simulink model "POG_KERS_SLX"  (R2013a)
settings: Solver=ode45  StartTime=0.0  StopTime=10.0  MaxStep=0.001  RelTol=1e-3
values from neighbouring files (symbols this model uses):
  b_1 = 0    [POG_KERS_Par_SLX_m.m]    (also in POG_KERS_SLX_m.m = 1)
  b_2 = 0    [POG_KERS_Par_SLX_m.m]    (also in POG_KERS_SLX_m.m = 1)
  b_3 = 0    [POG_KERS_Par_SLX_m.m]    (also in POG_KERS_SLX_m.m = 1)
  b_b = 0    [POG_KERS_Par_SLX_m.m]    (also in POG_KERS_SLX_m.m = 1)
  J_1 = 0.026*kg*meters^2    [POG_KERS_Par_SLX_m.m]    (also in POG_KERS_SLX_m.m = 13)
  J_2 = 0.675*kg*r_2^2    [POG_KERS_Par_SLX_m.m]    (also in POG_KERS_SLX_m.m = 1)
  J_3 = 100*J_2    [POG_KERS_Par_SLX_m.m]    (also in POG_KERS_SLX_m.m = 1)
  J_b = 1.0*kg*r_b^2    [POG_KERS_Par_SLX_m.m]    (also in POG_KERS_SLX_m.m = 1)
  K_1_2 = Inf    (= inf)    [POG_KERS_EQN_Reduced.m]    (also in POG_KERS_Par_SLX_m.m = 150*Newton/(0.2*mm); POG_KERS_SLX_m.m = 1)
  K_2_b = Inf    (= inf)    [POG_KERS_EQN_Reduced.m]    (also in POG_KERS_Par_SLX_m.m = 80*Newton/(0.2*mm); POG_KERS_SLX_m.m = 1)
  K_b_3 = Inf    (= inf)    [POG_KERS_EQN_Reduced.m]    (also in POG_KERS_Par_SLX_m.m = 80*Newton/(0.2*mm); POG_KERS_SLX_m.m = 1)
  P_1_6_0 = 0    [POG_KERS_SLX_m.m]
  P_2_0 = 2    [POG_KERS_SLX_m.m]
  P_2_3_0 = 0    [POG_KERS_SLX_m.m]
  P_9_0 = 0    [POG_KERS_SLX_m.m]
  r_1 = 17.2*mm    [POG_KERS_Par_SLX_m.m]    (also in POG_KERS_SLX_m.m = 1)
  r_2 = 51.5*mm    [POG_KERS_Par_SLX_m.m]    (also in POG_KERS_SLX_m.m = 1)
  r_2_t_h = r_a+r_b*sin(th_0)    [POG_KERS_Par_SLX_m.m]    (also in POG_KERS_SLX_m.m = 1)
  r_3_t_h = r_a-r_b*sin(th_0)    [POG_KERS_Par_SLX_m.m]    (also in POG_KERS_SLX_m.m = 1)
  r_b = 27.5*mm    [POG_KERS_Par_SLX_m.m]    (also in POG_KERS_SLX_m.m = 1)
  T_1_0 = 0*Nm    [POG_KERS_Par_SLX_m.m]    (also in POG_KERS_SLX_m.m = 0)
  Ts = Tfin/Nr_Ts_Points    (= 0.0015)    [POG_KERS_Par_SLX_m.m]    (also in POG_KERS_SLX_m.m = 0.005)
  x_1_3_0 = 0    [POG_KERS_Par_SLX_m.m]    (also in POG_KERS_SLX_m.m)
  x_2_0_0 = 0    [POG_KERS_Par_SLX_m.m]    (also in POG_KERS_SLX_m.m)
  x_6_0 = 0    [POG_KERS_Par_SLX_m.m]    (also in POG_KERS_SLX_m.m)

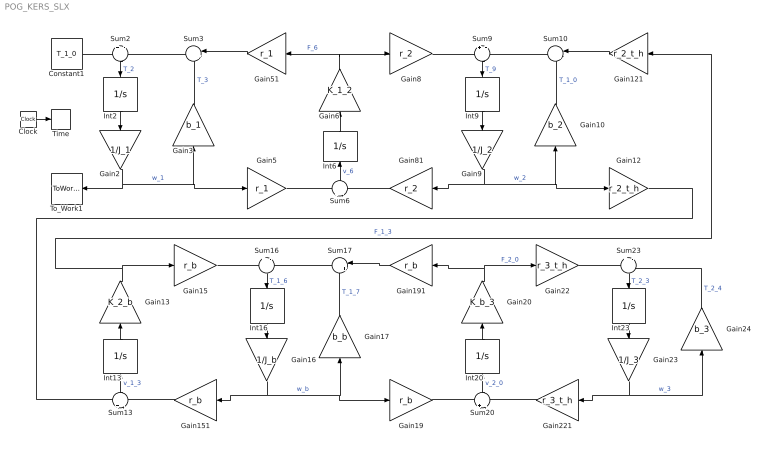
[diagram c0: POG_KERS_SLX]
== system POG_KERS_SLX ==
  Clock : Clock
  Constant1 : Constant  Value=T_1_0
  Gain10 : Gain  Gain=b_2  Multiplication=Matrix(K*u)
  Gain12 : Gain  Gain=r_2_t_h  Multiplication=Matrix(K*u)
  Gain121 : Gain  Gain=r_2_t_h  Multiplication=Matrix(K*u)
  Gain13 : Gain  Gain=K_2_b  Multiplication=Matrix(K*u)
  Gain{15,19,151,191} (4 alike) : Gain  Gain=r_b  Multiplication=Matrix(K*u)
  Gain16 : Gain  Gain=1/J_b  Multiplication=Matrix(K*u)
  Gain17 : Gain  Gain=b_b  Multiplication=Matrix(K*u)
  Gain2 : Gain  Gain=1/J_1  Multiplication=Matrix(K*u)
  Gain20 : Gain  Gain=K_b_3  Multiplication=Matrix(K*u)
  Gain22 : Gain  Gain=r_3_t_h  Multiplication=Matrix(K*u)
  Gain221 : Gain  Gain=r_3_t_h  Multiplication=Matrix(K*u)
  Gain23 : Gain  Gain=1/J_3  Multiplication=Matrix(K*u)
  Gain24 : Gain  Gain=b_3  Multiplication=Matrix(K*u)
  Gain3 : Gain  Gain=b_1  Multiplication=Matrix(K*u)
  Gain5 : Gain  Gain=r_1  Multiplication=Matrix(K*u)
  Gain51 : Gain  Gain=r_1  Multiplication=Matrix(K*u)
  Gain6 : Gain  Gain=K_1_2  Multiplication=Matrix(K*u)
  Gain8 : Gain  Gain=r_2  Multiplication=Matrix(K*u)
  Gain81 : Gain  Gain=r_2  Multiplication=Matrix(K*u)
  Gain9 : Gain  Gain=1/J_2  Multiplication=Matrix(K*u)
  Int13 : Integrator  InitialCondition=x_1_3_0
  Int16 : Integrator  InitialCondition=P_1_6_0
  Int2 : Integrator  InitialCondition=P_2_0
  Int20 : Integrator  InitialCondition=x_2_0_0
  Int23 : Integrator  InitialCondition=P_2_3_0
  Int6 : Integrator  InitialCondition=x_6_0
  Int9 : Integrator  InitialCondition=P_9_0
  Sum10 : Sum  Inputs=|++
  Sum{2,6,9,13,16,20,23} (7 alike) : Sum  Inputs=+|-
  Sum17 : Sum  Inputs=|++
  Sum3 : Sum  Inputs=|++
  Time : ToWorkspace  VariableName=t  SampleTime=Ts
  To_Work1 : ToWorkspace  VariableName=w_1_0  SampleTime=Ts
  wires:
  Constant1/1 -> Sum2/1
  Sum3/1 -> Sum2/2
  Gain2/1 -> To_Work1/1, Gain3/1, Gain5/1  "w_1"
  Sum2/1 -> Int2/1  "T_2"
  Int2/1 -> Gain2/1
  Gain51/1 -> Sum3/1
  Gain3/1 -> Sum3/2  "T_3"
  Gain5/1 -> Sum6/1
  Gain6/1 -> Gain51/1, Gain8/1  "F_6"
  Gain81/1 -> Sum6/2
  Sum6/1 -> Int6/1  "v_6"
  Int6/1 -> Gain6/1
  Gain8/1 -> Sum9/1
  Gain9/1 -> Gain81/1, Gain10/1, Gain12/1  "w_2"
  Sum10/1 -> Sum9/2
  Sum9/1 -> Int9/1  "T_9"
  Int9/1 -> Gain9/1
  Gain121/1 -> Sum10/1
  Gain10/1 -> Sum10/2  "T_1_0"
  Gain12/1 -> Sum13/1
  Gain13/1 -> Gain121/1, Gain15/1  "F_1_3"
  Gain151/1 -> Sum13/2
  Sum13/1 -> Int13/1  "v_1_3"
  Int13/1 -> Gain13/1
  Gain15/1 -> Sum16/1
  Gain16/1 -> Gain151/1, Gain17/1, Gain19/1  "w_b"
  Sum17/1 -> Sum16/2
  Sum16/1 -> Int16/1  "T_1_6"
  Int16/1 -> Gain16/1
  Gain191/1 -> Sum17/1
  Gain17/1 -> Sum17/2  "T_1_7"
  Gain19/1 -> Sum20/1
  Gain20/1 -> Gain191/1, Gain22/1  "F_2_0"
  Gain221/1 -> Sum20/2
  Sum20/1 -> Int20/1  "v_2_0"
  Int20/1 -> Gain20/1
  Gain22/1 -> Sum23/1
  Gain23/1 -> Gain221/1, Gain24/1  "w_3"
  Gain24/1 -> Sum23/2  "T_2_4"
  Sum23/1 -> Int23/1  "T_2_3"
  Int23/1 -> Gain23/1
  Clock/1 -> Time/1
